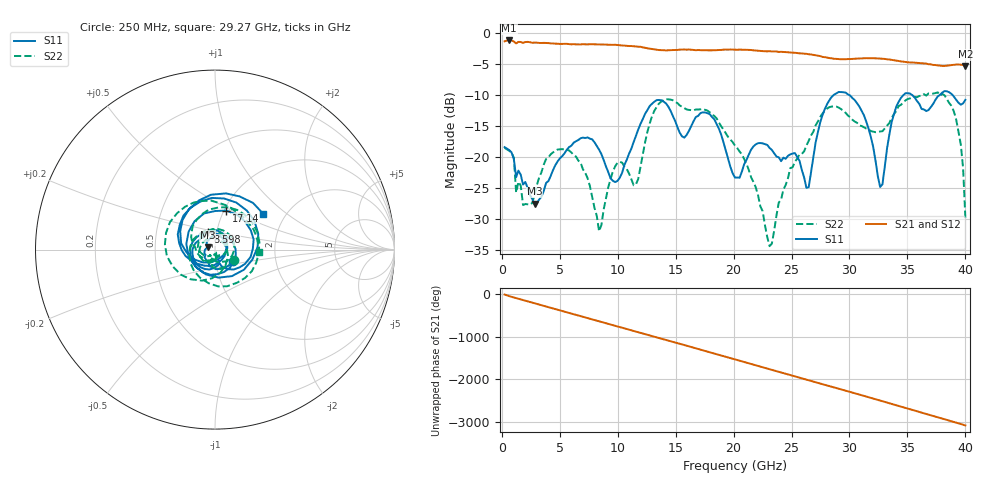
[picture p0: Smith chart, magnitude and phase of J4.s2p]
!Agilent Technologies,E8364B,MY43040528,A.07.50.67
!Agilent E8364B: A.07.50.67
!Date: Thursday, May 22, 2025 22:53:46
!Correction: S11(Full 2 Port(1,2))
!S21(Full 2 Port(1,2))
!S12(Full 2 Port(1,2))
!S22(Full 2 Port(1,2))
!S2P File: Measurements: S11, S21, S12, S22:
# Hz S  dB  R 50
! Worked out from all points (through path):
!   201 points, 250 MHz to 40 GHz, reference 50 ohm
!   highest |S21| = -1.20 dB at 647.5 MHz (marker M1); lowest = -5.3 dB at 40 GHz (marker M2)
!   group delay of S21, straight-line fit = 214 ps
!   lowest |S11| = -27.5 dB at 2.834 GHz (marker M3), VSWR 1.09, Z = 46.1 + j1.09 ohm
!   |S11| at or under -10 dB: start of sweep to 28.63 GHz; 29.99 GHz to 34.65 GHz (4.662 GHz wide, 14.4 % of centre); 35.42 GHz to 37.77 GHz (2.35 GHz wide, 6.42 % of centre)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
!   |S22| runs from -34.3 to -9.6 dB; largest |S21 - S12| = 0.008
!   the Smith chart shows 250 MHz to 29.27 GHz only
!   S11 on the Smith chart (normalised r, x): 250 MHz: 1.22, -0.16; 8.598 GHz: 0.91, +0.18; 17.14 GHz: 1.03, +0.47; 29.27 GHz: 1.55, +0.70
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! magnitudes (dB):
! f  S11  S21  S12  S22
! 250 MHz  -18.4  -1.3  -1.3  -18.5
! 647.5 MHz  -18.8  -1.2  -1.2  -19.0
! 1.84 GHz  -24.4  -1.6  -1.6  -27.7
! 2.834 GHz  -27.5  -1.5  -1.5  -26.0
! 4.821 GHz  -20.7  -1.7  -1.7  -18.8
! 7.008 GHz  -16.8  -1.8  -1.8  -21.9
! 8.598 GHz  -19.5  -1.8  -1.8  -30.9
! 9.989 GHz  -23.8  -1.9  -1.9  -20.9
! 11.58 GHz  -16.6  -2.2  -2.1  -24.4
! 13.57 GHz  -10.8  -2.7  -2.7  -11.4
! 17.14 GHz  -12.9  -2.8  -2.8  -12.3
! 20.12 GHz  -23.3  -2.7  -2.7  -18.1
! 23.11 GHz  -18.5  -2.9  -3.0  -34.3
! 26.29 GHz  -24.9  -3.3  -3.3  -18.1
! 26.88 GHz  -20.1  -3.5  -3.5  -15.9
! 29.27 GHz  -9.5  -4.2  -4.2  -12.2
! 31.25 GHz  -13.3  -4.1  -4.1  -15.2
! 32.65 GHz  -24.8  -4.1  -4.1  -15.9
! 33.44 GHz  -16.3  -4.3  -4.3  -14.5
! 38.21 GHz  -9.3  -5.3  -5.3  -10.0
! 39.6 GHz  -11.5  -5.1  -5.1  -17.9
! 40 GHz  -10.8  -5.3  -5.3  -29.9
